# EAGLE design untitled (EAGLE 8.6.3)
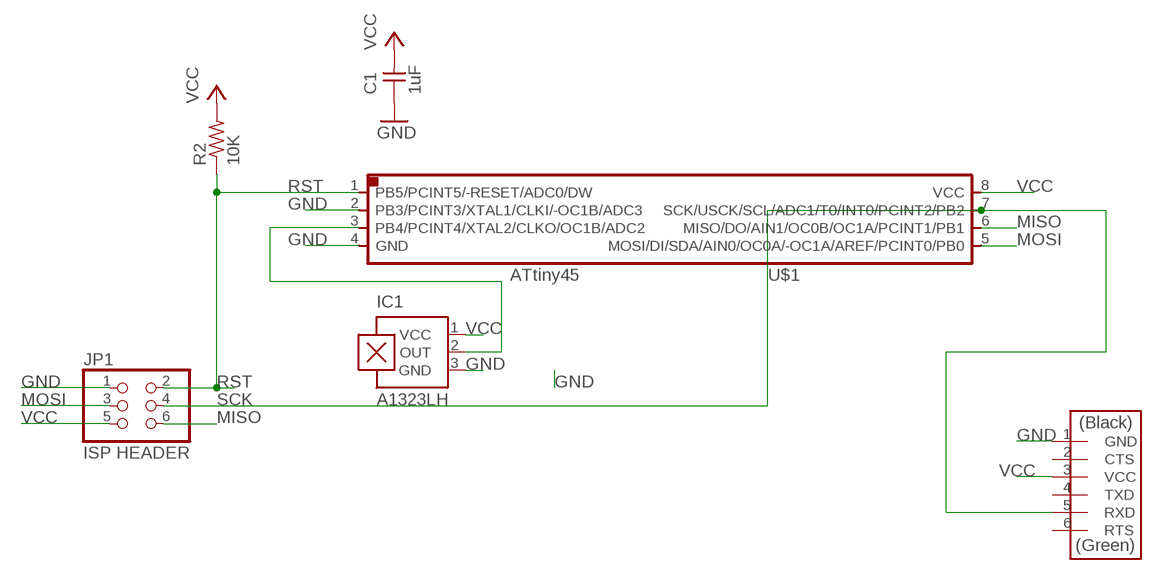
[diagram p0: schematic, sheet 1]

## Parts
C1  1uF  CAP-UNPOLARIZEDFAB  [C1206FAB]
IC1  A1323LH  [SOT23-W]
JP1  ISP HEADER  PINHD-2X3-SMD  [2X03SMD]
R2  10K  RES-US1206FAB  [R1206FAB]
U$1  ATTINY45SI  [SOIC8]
U$2  FTDI-SMD-HEADER  [1X06SMD]

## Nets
GND: C1.1 IC1.3(GND) JP1.1 U$1.2(PB3/PCINT3/XTAL1/CLKI/-OC1B/ADC3) U$1.4(GND) U$2.1(GND)
MISO: JP1.6 U$1.6(MISO/DO/AIN1/OC0B/OC1A/PCINT1/PB1)
MOSI: JP1.3 U$1.5(MOSI/DI/SDA/AIN0/OC0A/-OC1A/AREF/PCINT0/PB0)
N$1: IC1.2(OUT) U$1.3(PB4/PCINT4/XTAL2/CLKO/OC1B/ADC2)
RST: JP1.2 R2.1 U$1.1(PB5/PCINT5/-RESET/ADC0/DW)
SCK: JP1.4 U$1.7(SCK/USCK/SCL/ADC1/T0/INT0/PCINT2/PB2) U$2.5(RXD)
VCC: C1.2 IC1.1(VCC) JP1.5 R2.2 U$1.8(VCC) U$2.3(VCC)
Unconnected: U$2.2(CTS) U$2.4(TXD) U$2.6(RTS)

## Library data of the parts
C1 = fab:CAP-UNPOLARIZED
IC1 = allegro:A13*?: Linear Hall Effect Sensor ICs Continuous-Time Ratiometric High-Temperature Operation Programmable Linear with Analog Output A1302 -Replacement- UGN3503 Source: http://www.allegromicro.com/en/Products/Part_Numbers/1301/1301.pdf http://www.allegromicro.com/en/Products/Part_Numbers/1321/1321.pdf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; MF: ALLEGRO MICROSYSTEMS, INC.; MPN: A1323LLHLT-T; OC_FARNELL: 1651968; OC_NEWARK: 65K5152
JP1 = fab:PINHD-2X3-SMD: PIN HEADER
R2 = fab:RES-US: Resistor (US Symbol)
U$1 = fab:ATTINY45
U$2 = fab:FTDI-SMD-HEADER

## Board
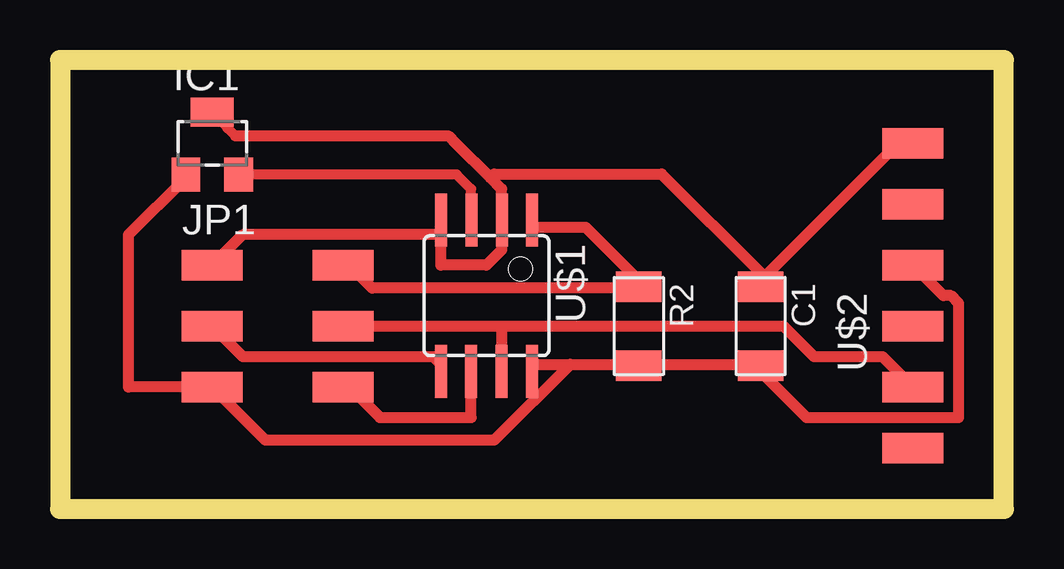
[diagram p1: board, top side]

Size 39.35 x 18.72 mm. Coordinates in mm from the lower left corner, seen from the top.
Outline: 0,0 39.35,0 39.35,18.72 0,18.72 0,0
Copper layers (1*16): Top 0.035mm / dielectric 1.5mm / Bottom 0.035mm
Design rules "default *": minimum track width 18mil, minimum drill 0.35mm, track to track 16mil, track to pad 16mil, pad to pad 16mil, via to via 6mil, smd to smd 16mil, copper to edge 40mil, drill to drill 6mil, minimum pad ring 10mil, minimum via ring 8mil, stop-mask expansion 4mil, vias tented up to drill 0mil, thermal gap 10mil

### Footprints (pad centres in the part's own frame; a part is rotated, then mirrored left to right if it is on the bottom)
C1206FAB = smd 1.27 x 1.905: 1 -1.651,0; 2 1.651,0
SOT23-W = smd 1.2 x 1.4: 1 -1.1,-1.3; 2 1.1,-1.3 | smd 1.8 x 1.2: 3 0,1.3
2X03SMD = smd 2.54 x 1.27: 1 -2.54,2.54; 2 2.92,2.54; 3 -2.54,0; 4 2.92,0; 5 -2.54,-2.54; 6 2.92,-2.54
R1206FAB = smd 1.27 x 1.905: 1 -1.651,0; 2 1.651,0
SOIC8 = smd 0.5 x 2.2: 1 -1.905,-3.154; 2 -0.645,-3.154; 3 0.625,-3.154; 4 1.895,-3.154; 5 1.905,3.154; 6 0.635,3.154; 7 -0.635,3.154; 8 -1.905,3.154
1X06SMD = smd 2.54 x 1.27: 1 0,6.35; 2 0,3.81; 3 0,1.27; 4 0,-1.27; 5 0,-3.81; 6 0,-6.35

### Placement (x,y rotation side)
C1  29.21,7.62 270 top
IC1  6.35,15.24 0 top
JP1  8.89,7.62 0 top
R2  24.13,7.62 270 top
U$1  17.78,8.89 180 top
U$2  35.56,8.89 0 top

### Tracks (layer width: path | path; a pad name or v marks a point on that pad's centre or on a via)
GND
  Top 0.406: IC1.3 6.98,15.91 6.98,15.88 7.3,15.56
  Top 0.457: U$2.1 34.92,15.24 29.21,9.53 C1.1 29.21,9.84 25.08,13.97 18.1,13.97 17.94,13.81 | 17.94,13.81 18.41,13.34 18.41,12.07 U$1.2 18.41,11.75 18.41,10.8 17.78,10.16 15.88,10.16 15.88,11.43 | 17.94,13.81 16.51,15.24 16.19,15.56 7.3,15.56 | 15.88,11.43 15.88,11.75 U$1.4 15.88,11.43 | JP1.1 7.62,11.43 15.88,11.43
MISO
  Top 0.457: U$1.6 17.14,3.81 13.33,3.81 12.06,5.08 JP1.6
MOSI
  Top 0.457: JP1.3 7.62,6.35 15.56,6.35 15.88,6.03 U$1.5
N$1
  Top 0.406: U$1.3 17.14,12.05 17.14,13.34 16.54,13.94 IC1.2
RST
  Top 0.457: U$1.1 19.69,11.75 21.91,11.75 24.13,9.53 R2.1 24.13,9.21 13.02,9.21 12.06,10.16 JP1.2
SCK
  Top 0.457: 18.41,7.62 U$1.7 | JP1.4 18.41,7.62 | U$2.5 34.29,6.35 31.43,6.35 30.16,7.62 18.41,7.62
VCC
  Top 0.406: 5.25,13.82 IC1.1
  Top 0.457: 21.27,6.03 19.69,6.03 U$1.8 | 21.27,6.03 24.13,6.03 | 24.13,6.03 29.21,6.03 C1.2 29.21,5.72 31.11,3.81 37.47,3.81 37.47,8.57 37.15,8.89 36.83,8.89 U$2.3 | 24.13,6.03 R2.2 | 21.27,6.03 18.1,2.86 8.57,2.86 JP1.5 2.86,5.08 2.86,11.43 5.25,13.82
